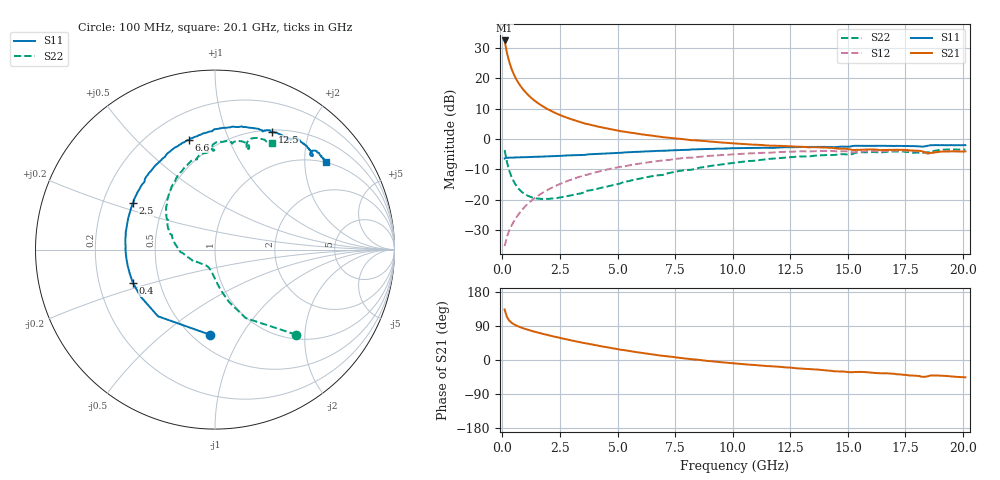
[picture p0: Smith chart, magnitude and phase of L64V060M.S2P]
!  Infineon Technologies AG
! BFR380L3 , PF131585-7, No.6, Th 09.10.01, soldered on pcb-board, measured with PP GSG850
!  Vce=4.0 V,  Ic=60.0 mA
! Common Emitter S-Parameters:  15. November 2001
#  GHz  S  MA  R  50
! f  S11  S21  S12  S22
! GHz  Mag  Ang  Mag  Ang  Mag  Ang  Mag  Ang
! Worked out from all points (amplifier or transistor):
!   201 points, 100 MHz to 20.1 GHz, reference 50 ohm
!   highest |S21| = 32.5 dB at 100 MHz (marker M1)
!   |S21| within 3 dB of that: start of sweep to 174.1 MHz
!   unconditionally stable (mu >= 1): 851.3 MHz to 4.221 GHz; 18.38 GHz to 18.5 GHz
!   at 3.4 GHz: K = 1.02, MAG = 8.1 dB, |S12| = -12.4 dB
!   at 10.1 GHz: K = 0.95, MSG = 1.8 dB, |S12| = -5.0 dB
!   at 20.1 GHz: K = 0.99, MSG = 0.0 dB, |S12| = -4.1 dB
!   S11 on the Smith chart (normalised r, x): 100 MHz: 0.61, -0.74; 400 MHz: 0.35, -0.17; 2.5 GHz: 0.33, +0.24; 6.6 GHz: 0.36, +0.73; 12.5 GHz: 0.52, +1.47; 20.1 GHz: 0.99, +2.55
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0.1  0.4758 -93.0  42.21 133.4  0.01697 60.3  0.656 -46.3
0.2  0.4888 -130.5  26.49 113.5  0.02395 58.1  0.4176 -65.9
0.3  0.4904 -147.8  18.74 104.2  0.03084 60.1  0.3008 -75.1
0.4  0.4936 -158.1  14.38 98.4  0.03693 62.6  0.2363 -80.9
0.5  0.4934 -164.5  11.63 94.3  0.04332 65.2  0.1968 -85.3
0.6  0.4947 -169.6  9.753 91.1  0.04999 66.6  0.1705 -88.7
0.7  0.4959 -173.7  8.41 88.4  0.05669 67.7  0.1519 -91.9
0.8  0.497 -176.8  7.384 86.0  0.06365 68.6  0.1384 -94.7
1  0.4988 177.6  5.945 81.8  0.07737 69.4  0.121 -99.8
1.3  0.5037 171.0  4.61 76.4  0.09813 69.4  0.1081 -107.1
1.6  0.5086 165.2  3.776 71.4  0.1188 68.7  0.1029 -113.9
2  0.5157 158.3  3.055 65.4  0.1464 67.0  0.1024 -122.6
2.5  0.5257 150.6  2.485 58.3  0.1804 64.2  0.1077 -132.6
3.5  0.5451 136.7  1.838 45.3  0.2469 57.9  0.1292 -149.2
4.9  0.5847 120.2  1.4 29.7  0.3333 48.4  0.1758 -172.4
6.6  0.6288 103.2  1.119 13.9  0.425 36.4  0.2464 164.6
6.8  0.6347 101.3  1.092 12.3  0.4351 34.8  0.2521 162.1
10.1  0.7007 76.9  0.8414 -9.1  0.5592 12.7  0.4055 129.0
12.5  0.7288 64.1  0.7555 -20.3  0.6163 -2.3  0.4978 107.7
13.5  0.7367 59.6  0.7301 -24.6  0.6268 -8.4  0.5242 100.5
16.8  0.7686 47.4  0.6605 -35.4  0.6331 -24.6  0.6155 78.8
20.1  0.7888 38.2  0.6242 -45.8  0.6253 -38.4  0.672 62.1
